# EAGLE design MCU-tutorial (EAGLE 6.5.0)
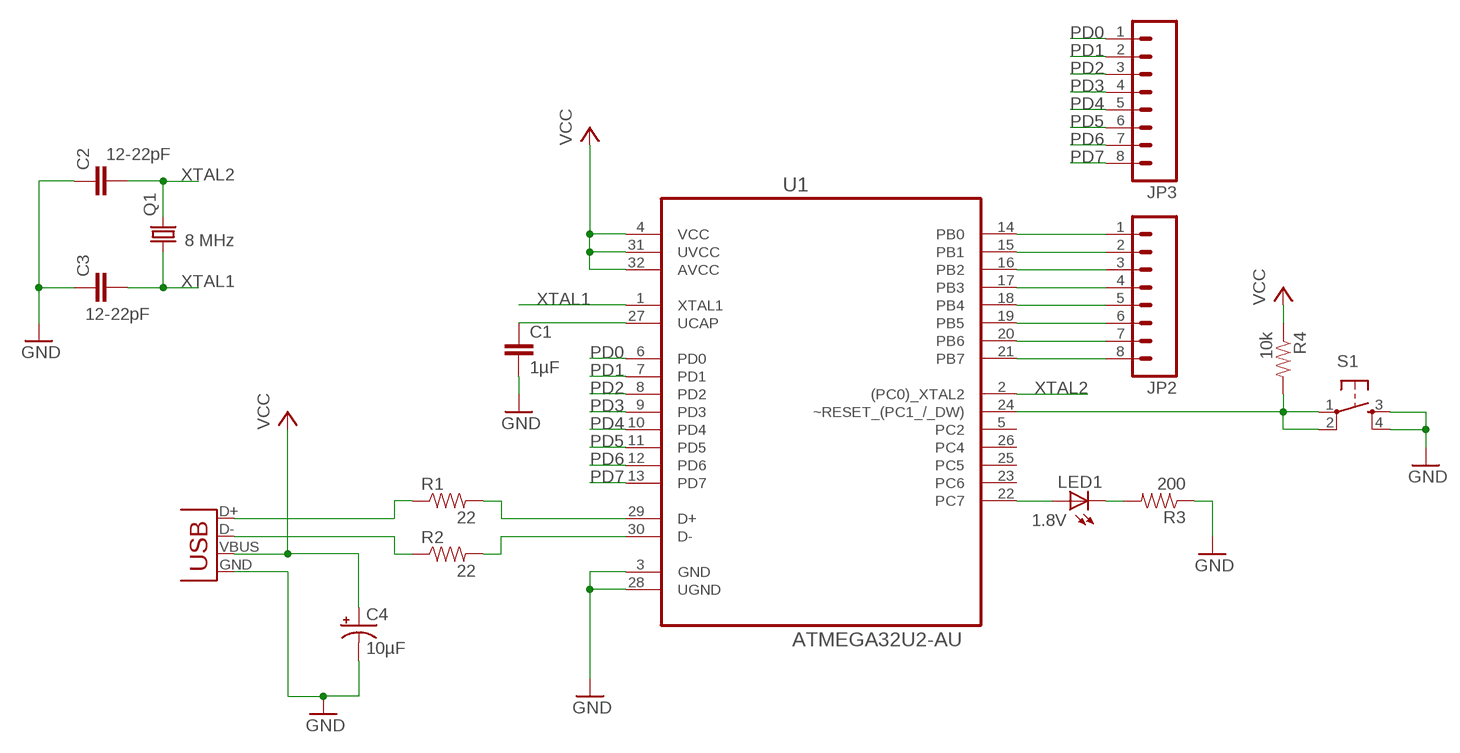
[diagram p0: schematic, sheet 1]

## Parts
C1  1µF  CAP1206  [1206]
C2  12-22pF  CAP1206  [1206]
C3  12-22pF  CAP1206  [1206]
C4  10µF  CAP_POLPTH4  [CPOL-RADIAL-1000UF-25V]
JP1  USB-B  USBPTH  [USB-B-PTH]
JP2  M08LOCK_LONGPADS  [1X08_LOCK_LONGPADS]
JP3  M08LOCK_LONGPADS  [1X08_LOCK_LONGPADS]
LED1  1.8V  LED-5MM  [LED-5MM]
Q1  8 MHz  CRYSTALHC49UP  [HC49UP]
R1  22  RESISTOR1206  [1206]
R2  22  RESISTOR1206  [1206]
R3  200  RESISTOR1206  [1206]
R4  10k  RESISTOR1206  [1206]
S1  TAC_SWITCHPTH  [TACTILE-PTH]
U1  ATMEGA32U2-AU  [QFP80P900X900X120-32N]

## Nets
GND: C1.2 C2.1 C3.1 C4.2(-) JP1.GND R3.1 S1.3 S1.4 U1.3(GND) U1.28(UGND)
N$1: JP1.D+ R1.1
N$2: JP1.D- R2.1
N$3: R2.2 U1.30(D-)
N$4: R1.2 U1.29(D+)
N$5: R4.2 S1.1 S1.2 U1.24(~RESET_(PC1_/_DW))
N$6: LED1.A U1.22(PC7)
N$7: C1.1 U1.27(UCAP)
N$8: LED1.K(C) R3.2
PB0: JP2.1 U1.14(PB0)
PB1: JP2.2 U1.15(PB1)
PB2: JP2.3 U1.16(PB2)
PB3: JP2.4 U1.17(PB3)
PB4: JP2.5 U1.18(PB4)
PB5: JP2.6 U1.19(PB5)
PB6: JP2.7 U1.20(PB6)
PB7: JP2.8 U1.21(PB7)
PD0: JP3.1 U1.6(PD0)
PD1: JP3.2 U1.7(PD1)
PD2: JP3.3 U1.8(PD2)
PD3: JP3.4 U1.9(PD3)
PD4: JP3.5 U1.10(PD4)
PD5: JP3.6 U1.11(PD5)
PD6: JP3.7 U1.12(PD6)
PD7: JP3.8 U1.13(PD7)
VCC: C4.1(+) JP1.VBUS R4.1 U1.4(VCC) U1.31(UVCC) U1.32(AVCC)
XTAL1: C3.2 Q1.1 U1.1(XTAL1)
XTAL2: C2.2 Q1.2 U1.2((PC0)_XTAL2)
Unconnected: U1.5(PC2) U1.23(PC6) U1.25(PC5) U1.26(PC4)

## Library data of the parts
C1-C3 = SparkFun:CAP: Capacitor
C4 = SparkFun:CAP_POL: Capacitor Polarized
JP1 = SparkFun-Connectors:USB: USB Connectors USB-B-PTH is fully proven SKU : PRT-00139/CONN-08278 USB-miniB is fully proven SKU : PRT-00587 USB-A-PCB is untested. USB-A-H is throughly reviewed, but untested. Spark Fun Electronics SKU : PRT-00437 USB-B-SMT is throughly reviewed, but untested. Needs silkscreen touching up.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; PROD_ID: CONN-08278
JP2 JP3 = SparkFun-Connectors:M08: Header 8 Standard 8-pin 0.1" header. Use with straight break away headers (SKU : PRT-00116), right angle break away headers (PRT-00553), swiss pins (PRT-00743), machine pins (PRT-00117), and female headers (PRT-00115).
LED1 = dp_devices:LED: Light Emitting Diode
Q1 = crystal:CRYSTAL: CRYSTAL; OC_FARNELL: unknown; OC_NEWARK: unknown
R1-R4 = SparkFun:RESISTOR: Resistor
S1 = SparkFun:TAC_SWITCH: Momentary Switch Button commonly used for reset or general input. Spark Fun Electronics SKU : COM-00097
U1 = Atmel-ATMEGA32U2-AU:ATMEGA32U2-AU; DESCRIPTION: 8-bit Microcontroller with ISP Flash and USB Controller; MPN: ATMEGA32U2-AU; OC_FARNELL: 1748524; OC_NEWARK: 26R5632; PACKAGE: TQFP-32; SUPPLIER: Atmel

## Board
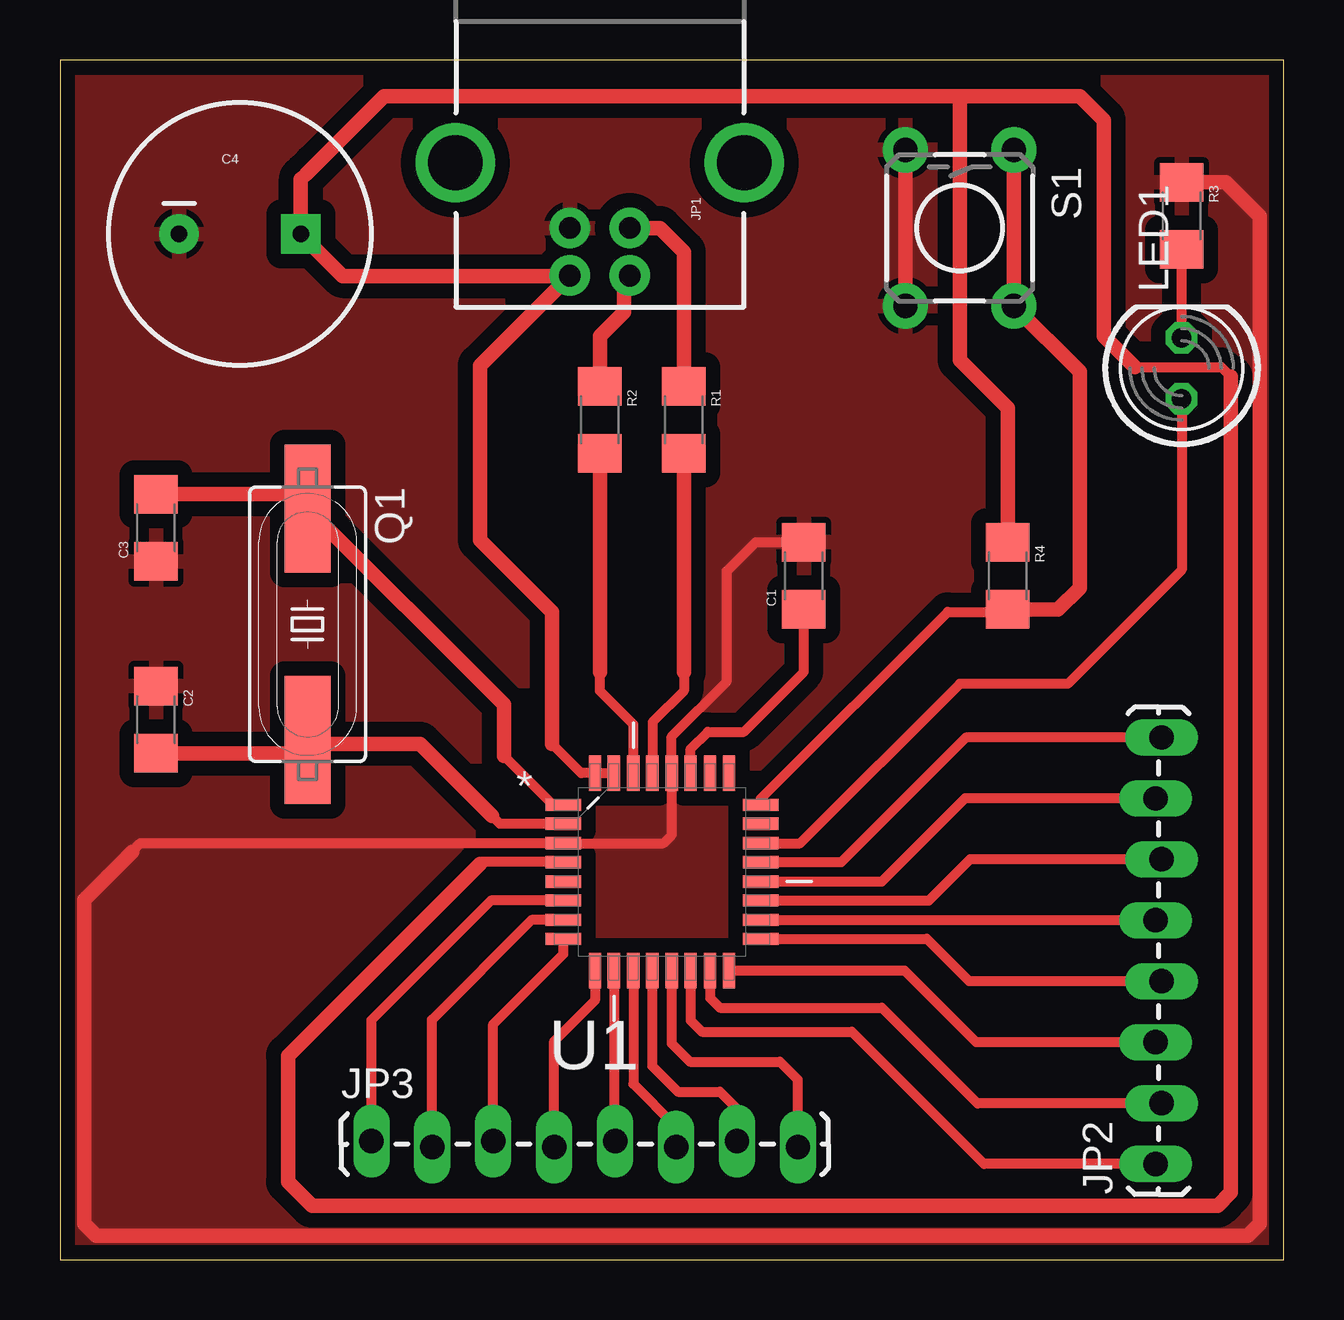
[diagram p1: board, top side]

Size 51 x 50 mm. Coordinates in mm from the lower left corner, seen from the top.
Outline: 0,0 51,0 51,50 0,50 0,0
Copper layers (1*16): Top 0.035mm / dielectric 1.5mm / Bottom 0.035mm
Design rules "SeeedStudio_2layer_DRU_no_angle_20140221": minimum track width 6mil, minimum drill 12mil, track to track 6mil, track to pad 6mil, pad to pad 6mil, via to via 6mil, smd to smd 0mil, copper to edge 10mil, drill to drill 10mil, minimum pad ring 10mil, minimum via ring 6mil, stop-mask expansion 2mil, vias tented up to drill 100mil, thermal gap 10mil

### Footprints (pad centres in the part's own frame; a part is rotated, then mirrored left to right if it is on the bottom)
1206 = smd 1.6 x 1.8: 1 -1.4,0; 2 1.4,0
CPOL-RADIAL-1000UF-25V = drill 0.7 pad 1.651 square: 1 2.54,0 | drill 0.7 pad 1.651: 2 -2.54,0
USB-B-PTH = drill 0.914 pad 1.676: D+ 0,1.25; D- 1.981,1.25; GND 0,-1.25; VBUS 1.981,-1.25 | drill 2.286: S1 -2.718,-6.02; S2 -2.718,6.02
1X08_LOCK_LONGPADS = drill 1.016 long: 1 0,0.127; 2 2.54,-0.127; 3 5.08,0.127; 4 7.62,-0.127; 5 10.16,0.127; 6 12.7,-0.127; 7 15.24,0.127; 8 17.78,-0.127
LED-5MM = drill 0.813 octagon: A -1.27,0; K 1.27,0
HC49UP = smd 5.334 x 1.93: 1 -4.826,0; 2 4.826,0
TACTILE-PTH = drill 1.016 pad 1.88: 1 -3.251,2.261; 2 3.251,2.261; 3 -3.251,-2.261; 4 3.251,-2.261
QFP80P900X900X120-32N = smd 1.473 x 0.508: 1 -4.115,2.794; 2 -4.115,2.007; 3 -4.115,1.194; 4 -4.115,0.406; 5 -4.115,-0.406; 6 -4.115,-1.194; 7 -4.115,-2.007; 8 -4.115,-2.794; 17 4.115,-2.794; 18 4.115,-2.007; 19 4.115,-1.194; 20 4.115,-0.406; 21 4.115,0.406; 22 4.115,1.194; 23 4.115,2.007; 24 4.115,2.794 | smd 0.508 x 1.473: 9 -2.794,-4.115; 10 -2.007,-4.115; 11 -1.194,-4.115; 12 -0.406,-4.115; 13 0.406,-4.115; 14 1.194,-4.115; 15 2.007,-4.115; 16 2.794,-4.115; 25 2.794,4.115; 26 2.007,4.115; 27 1.194,4.115; 28 0.406,4.115; 29 -0.406,4.115; 30 -1.194,4.115; 31 -2.007,4.115; 32 -2.794,4.115

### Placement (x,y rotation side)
C1  31,28.5 90 top
C2  4,22.5 270 top
C3  4,30.5 90 top
C4  7.5,42.75 0 top
JP1  22.5,43 270 top
JP2  45.79,3.98 90 top
JP3  12.98,4.81 0 top
LED1  46.75,37.15 90 top
Q1  10.32,26.48 270 top
R1  26,35 270 top
R2  22.5,35 270 top
R3  46.75,43.5 270 top
R4  39.5,28.5 270 top
S1  37.5,43 270 top
U1  25.09,16.16 0 top

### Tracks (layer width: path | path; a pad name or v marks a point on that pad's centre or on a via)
GND
  Top 0.406: C1.2 29,29.9 27.8,28.7 27.8,24.1 25.5,21.8 U1.28 25.5,17.7 25.15,17.35 U1.3 3.35,17.35 3,17
  Top 0.61: S1.3 S1.4 | R3.1 48.6,44.9 50,43.5 50,1.5 49.5,1 1.5,1 1,1.5 1,15 3,17
  pour Top (isolate 0.61): 0,50 51,50 51,0 0,0
N$1
  Top 0.61: R1.1 26,42 25,43 JP1.D+
N$2
  Top 0.61: R2.1 22.5,38.5 23.5,39.5 23.5,40.77 JP1.D-
N$3
  Top 0.406: U1.30 23.9,22.3 22.5,23.7 22.5,24.5
  Top 0.61: 22.5,24.5 R2.2
N$4
  Top 0.406: 26,24.5 26,23.7 24.7,22.4 24.7,20.29 U1.29
  Top 0.61: 26,24.5 R1.2
N$5
  Top 0.406: U1.24 29.2,19.2 37,27 39.4,27 R4.2
  Top 0.61: S1.1 S1.2 42.5,37.01 42.5,28 41.6,27.1 R4.2
N$6
  Top 0.406: U1.22 30.85,17.35 37.5,24 42,24 46.75,28.75 LED1.A
N$7
  Top 0.406: C1.1 31,24.5 28.5,22 27,22 26.28,21.28 U1.27
N$8
  Top 0.406: LED1.K R3.2
PB0
  Top 0.406: U1.14 26.28,9.97 26.75,9.5 33,9.5 38.52,3.98 JP2.1
PB1
  Top 0.406: U1.15 27.1,10.9 27.5,10.5 34.25,10.5 38.25,6.5 38.27,6.52 JP2.2
PB2
  Top 0.406: U1.16 35.2,12.04 38.19,9.06 JP2.3
PB3
  Top 0.406: U1.17 36.13,13.37 37.9,11.6 JP2.4
PB4
  Top 0.406: U1.18 45.65,14.15 JP2.5
PB5
  Top 0.406: U1.19 36.22,14.97 37.93,16.68 JP2.6
PB6
  Top 0.406: U1.20 34.25,15.75 37.72,19.22 JP2.7
PB7
  Top 0.406: U1.21 32.57,16.57 37.76,21.76 JP2.8
PD0
  Top 0.406: U1.6 17.97,14.97 12.98,9.98 JP3.1
PD1
  Top 0.406: U1.7 19.65,14.15 15.5,10 15.52,9.98 JP3.2
PD2
  Top 0.406: U1.8 20.98,12.72 18.06,9.81 JP3.3
PD3
  Top 0.406: U1.9 22.3,10.8 20.6,9.1 JP3.4
PD4
  Top 0.406: U1.10 23.08,4.99 JP3.5
PD5
  Top 0.406: U1.11 23.9,7.32 25.68,5.53 JP3.6
PD6
  Top 0.406: U1.12 24.68,8.07 25.75,7 27.5,7 28.22,6.28 JP3.7
PD7
  Top 0.406: U1.13 25.5,9 26.25,8.25 30,8.25 30.76,7.49 JP3.8
VCC
  Top 0.406: 20.5,21.5 21.73,20.27 U1.32 U1.31 | U1.4 17.57,16.57 17.5,16.5 | 44.8,37.2 48.4,37.2 48.8,36.8
  Top 0.61: 20.5,21.5 20.5,27 17.5,30 17.5,37.27 JP1.VBUS 21.23,41 11.79,41 C4.1 10.04,45.04 10.25,45.25 10.62,45.62 13.5,48.5 37.5,48.5 | R4.1 39.5,35.5 37.5,37.5 37.5,48.5 | 37.5,48.5 42.5,48.5 43.5,47.5 43.5,38.5 44.8,37.2 | 17.5,16.5 9.5,8.5 9.5,3.25 10.5,2.25 48.25,2.25 48.8,2.8 48.8,36.8
XTAL1
  Top 0.406: U1.1 20.55,18.95 18.5,21
  Top 0.61: 18.5,21 18.5,23.13 Q1.1 9.73,31.9 C3.2
XTAL2
  Top 0.406: U1.2 18.33,18.17 18,18.5
  Top 0.61: 18,18.5 15,21.5 10.47,21.5 Q1.2 9.77,21.1 C2.2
